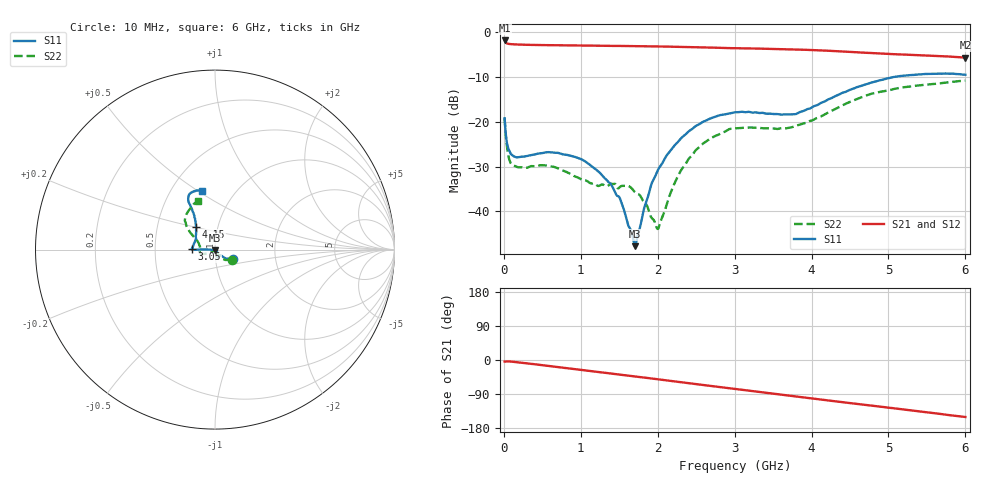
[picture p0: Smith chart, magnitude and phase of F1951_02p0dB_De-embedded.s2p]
! Integrated Device Technology
! Corporate Headquarters
! 6024 Silver Creek Valley Road
! San Jose, CA 95138  USA
! Phone:  1-408-284-8200
! Toll Free:  1-800-223-1366
! Webpage:  http://www.idt.com/
! Timing and RF Division
! 515 Groton Road, Suite 102
! Westford, MA 01886-6024
! Device:  F1951
! Description: 6-bit 0.5 dB Digital Step Attenuator
! Frequency:  100.0 -  4000.00 MHz
! Package:  4x4 mm Thin QFN Plastic Package: 24 pin
! Ports:  2 RF, 6 DC
!  Pin  1  = NC
!  Pin  2  = RF1  =  Port 1
!  Pin  3  = GND
!  Pin  4  = NC
!  Pin  5  = Serial Data Out (SDO)
!  Pin  6  = NC
!  Pin  7  = Reset Bar ( RSTb)
!  Pin  8  = Clock (CLK)
!  Pin  9  = Chip Select Bar (CSb)
!  Pin 10  = NC
!  Pin 11  = Serial Data In (SDI)
!  Pin 12  = NC
!  Pin 13  = NC
!  Pin 14  = VDD
!  Pin 15  = NC
!  Pin 16  = GND
!  Pin 17  = RF2  =  Port 2
!  Pin 18  = NC
!  Pin 19  = GND
!  Pin 20  = GND
!  Pin 21  = GND
!  Pin 22  = GND
!  Pin 23  = GND
!  Pin 24  = GND
! State:  4
! Atten State:  2.0 dB
! Voltage:  +3.30 Volts
! Current:  0.472 mA
! Data:  The device was measured on a F195X evaluation board which has
!  individual transmission lines to the RF pins.  Data was collected
!  de-embedded using a Automatic Fixture Removal [AFR] (Keysight Technologies).
!  The reference plane is the edge of the package pin.
! Misc:  Lot Code  1225BCA
!  Action Tracker AT0399
! Date Measured:  2018-09-13
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# GHz S dB R 50
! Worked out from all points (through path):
!   600 points, 10 MHz to 6 GHz, reference 50 ohm
!   highest |S21| = -1.83 dB at 10 MHz (marker M1); lowest = -5.7 dB at 6 GHz (marker M2)
!   group delay of S21, straight-line fit = 69.2 ps
!   lowest |S11| = -47.7 dB at 1.7 GHz (marker M3), VSWR 1.01, Z = 49.9 - j0.392 ohm
!   |S11| at or under -10 dB: start of sweep to 5.065 GHz
!   |S22| runs from -43.9 to -10.8 dB; largest |S21 - S12| = 0.0009
!   S11 on the Smith chart (normalised r, x): 10 MHz: 1.21, -0.12; 3.05 GHz: 0.77, +0.00; 4.15 GHz: 0.78, +0.21; 6 GHz: 0.71, +0.52
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0.01  -19.20 -27.2  -1.83 -3.9  -1.83 -3.9  -19.14 -31.5
0.07  -26.37 -44.7  -2.62 -3.9  -2.62 -3.9  -28.41 -55.4
0.12  -27.59 -49.6  -2.69 -4.7  -2.69 -4.7  -29.73 -59.8
0.63  -26.82 -72.5  -2.89 -16.8  -2.89 -16.8  -29.97 -74.9
1.01  -28.36 -63.6  -2.98 -26.1  -2.98 -26.1  -32.87 -50.6
1.4  -34.13 -49.7  -3.03 -35.7  -3.03 -35.7  -33.83 -6.0
1.52  -37.58 -48.4  -3.06 -38.6  -3.06 -38.6  -34.39 3.8
1.7  -47.75 -106.7  -3.09 -43.2  -3.09 -43.2  -35.62 5.7
1.73  -46.04 -138.1  -3.09 -44.0  -3.10 -44.0  -36.03 2.7
1.91  -34.39 -175.5  -3.14 -48.5  -3.15 -48.5  -41.16 -19.1
2.01  -30.52 179.9  -3.17 -51.1  -3.17 -51.1  -43.78 -74.2
2.23  -25.06 179.5  -3.24 -56.7  -3.24 -56.7  -33.29 -139.0
2.41  -22.02 179.5  -3.30 -61.3  -3.31 -61.3  -28.11 -147.9
2.66  -19.44 -179.7  -3.40 -67.7  -3.41 -67.7  -23.98 -157.6
3.01  -17.86 -179.9  -3.55 -76.3  -3.56 -76.3  -21.44 -167.4
3.05  -17.84 179.4  -3.57 -77.2  -3.57 -77.2  -21.41 -168.3
3.76  -18.31 151.3  -3.84 -95.2  -3.84 -95.2  -21.11 166.0
4.01  -16.72 135.9  -3.97 -101.5  -3.97 -101.5  -19.66 156.0
4.15  -15.59 129.7  -4.07 -105.0  -4.08 -105.0  -18.55 151.9
4.68  -11.76 119.7  -4.56 -117.9  -4.56 -117.9  -14.30 142.6
5.01  -10.22 118.9  -4.86 -125.9  -4.86 -125.9  -12.95 137.2
6  -9.48 102.2  -5.65 -150.4  -5.65 -150.4  -10.80 109.6
